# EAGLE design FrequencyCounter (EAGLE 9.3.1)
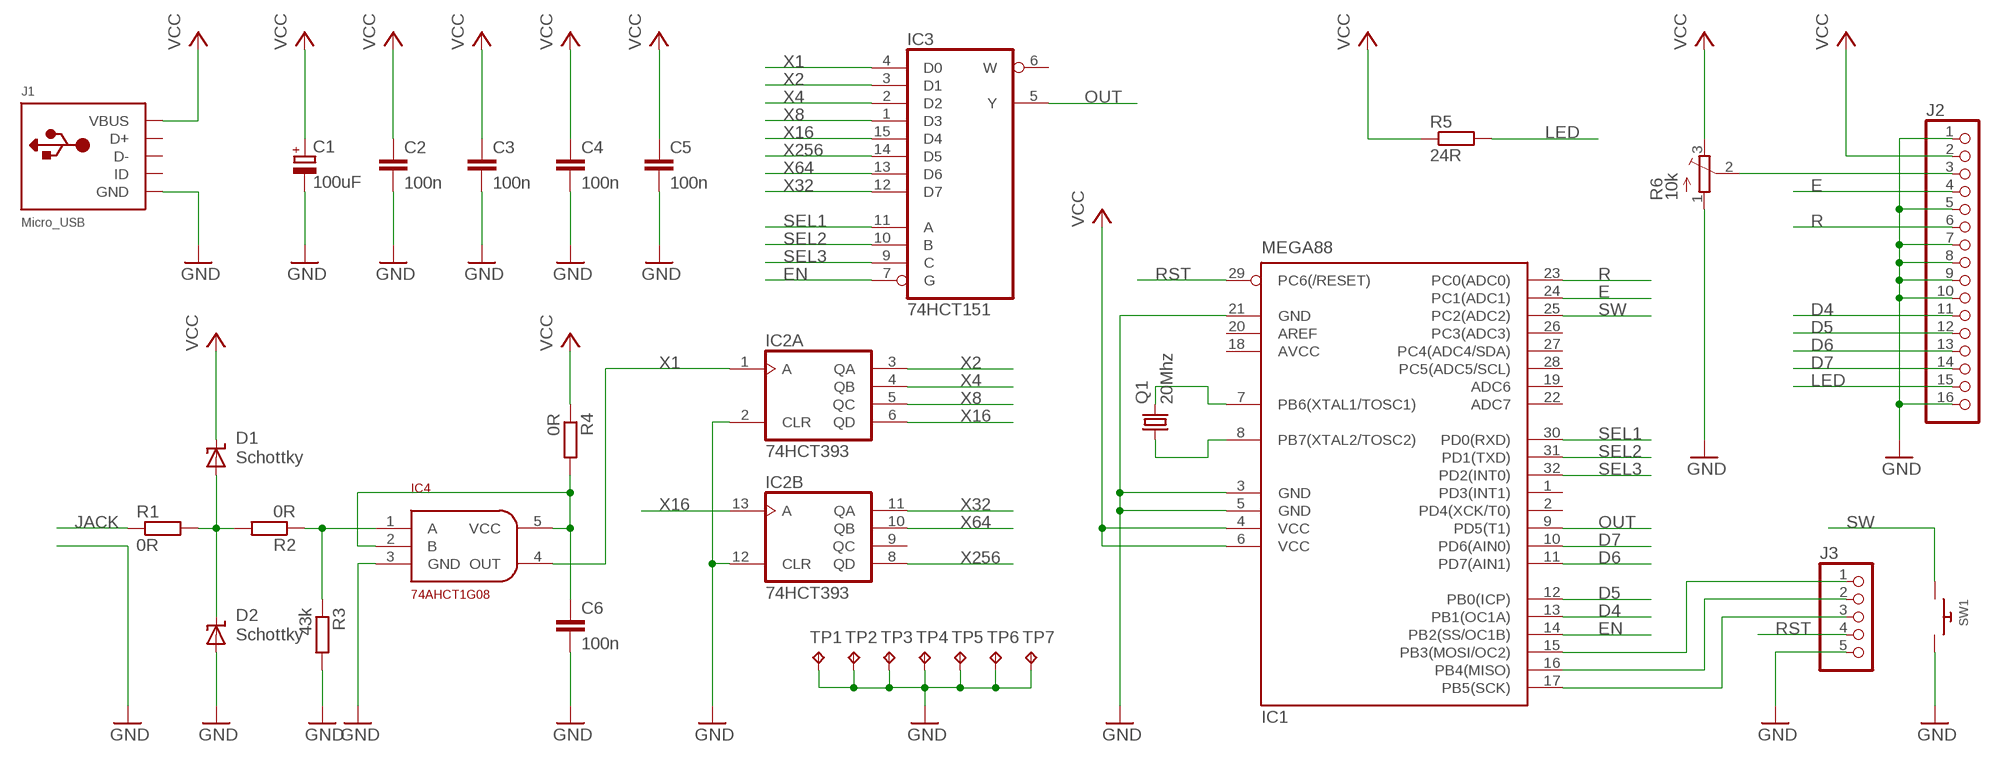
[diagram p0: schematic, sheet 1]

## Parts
C1  100uF  CPOL-EU153CLV-0605  [153CLV-0605]
C2  100n  C-EUC1206  [C1206]
C3  100n  C-EUC1206  [C1206]
C4  100n  C-EUC1206  [C1206]
C5  100n  C-EUC1206  [C1206]
C6  100n  C-EUC1206  [C1206]
D1  Schottky  SUPPRESSOR-SMBJ  [SMBJ]
D2  Schottky  SUPPRESSOR-SMBJ  [SMBJ]
IC1  MEGA88  MEGA8-AI  [TQFP32-08]
IC2  74HCT393  74AC393D  [SO14]
IC3  74HCT151  74AC151D  [SO16]
IC4  74AHCT1G08  [SOT-23-5]
J1  Micro_USB  USBMINIB  [USB-MINIB]
J2  PINHD-1X16  [1X16]
J3  PINHD-1X5  [1X05]
Q1  20Mhz  CSM-7X-DU  [CSM-7X-DU]
R1  0R  R-EU_M1206  [M1206]
R2  0R  R-EU_M1206  [M1206]
R3  43k  R-EU_M1206  [M1206]
R4  0R  R-EU_M1206  [M1206]
R5  24R  R-EU_M1206  [M1206]
R6  10k  TRIM_EU-3223G  [3223G]
SW1  SWITCH_PUSHBUTTONC&K_KSS  [BTN_CK_KSS]
TP1  TPPAD1-13  [P1-13]
TP2  TPPAD1-13  [P1-13]
TP3  TPPAD1-13  [P1-13]
TP4  TPPAD1-13  [P1-13]
TP5  TPPAD1-13  [P1-13]
TP6  TPPAD1-13  [P1-13]
TP7  TPPAD1-13  [P1-13]

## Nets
D4: IC1.13(PB1(OC1A)) J2.11
D5: IC1.12(PB0(ICP)) J2.12
D6: IC1.11(PD7(AIN1)) J2.13
D7: IC1.10(PD6(AIN0)) J2.14
E: IC1.24(PC1(ADC1)) J2.4
EN: IC1.14(PB2(SS/OC1B)) IC3.7(G)
GND: C1.- C2.2 C3.2 C4.2 C5.2 C6.2 D2.A IC1.3(GND) IC1.5(GND) IC1.21(GND) IC2.2(A:CLR) IC2.12(B:CLR) IC4.3(GND) J1.GND J2.1 J2.5 J2.7 J2.8 J2.9 J2.10 J2.16 J3.5 R3.2 R6.1(A) SW1.P$2 TP1.TP TP2.TP TP3.TP TP4.TP TP5.TP TP6.TP TP7.TP
JACK: R1.1
LED: J2.15 R5.2
N$1: IC1.17(PB5(SCK)) J3.3
N$2: D1.A D2.C R1.2 R2.2
N$3: IC4.1(A) R2.1 R3.1
N$4: IC1.16(PB4(MISO)) J3.2
N$5: IC1.15(PB3(MOSI/OC2)) J3.1
N$6: IC1.8(PB7(XTAL2/TOSC2)) Q1.1
N$7: IC1.7(PB6(XTAL1/TOSC1)) Q1.2
N$8: J2.3 R6.2(S)
N$10: C6.1 IC4.2(B) IC4.5(VCC) R4.2
OUT: IC1.9(PD5(T1)) IC3.5(Y)
R: IC1.23(PC0(ADC0)) J2.6
RST: IC1.29(PC6(/RESET)) J3.4
SEL1: IC1.30(PD0(RXD)) IC3.11(A)
SEL2: IC1.31(PD1(TXD)) IC3.10(B)
SEL3: IC1.32(PD2(INT0)) IC3.9(C)
SW: IC1.25(PC2(ADC2)) SW1.P$1
VCC: C1.+ C2.1 C3.1 C4.1 C5.1 D1.C IC1.4(VCC) IC1.6(VCC) J1.VBUS J2.2 R4.1 R5.1 R6.3(E)
X1: IC2.1(A:A) IC3.4(D0) IC4.4(OUT)
X2: IC2.3(A:QA) IC3.3(D1)
X4: IC2.4(A:QB) IC3.2(D2)
X8: IC2.5(A:QC) IC3.1(D3)
X16: IC2.6(A:QD) IC2.13(B:A) IC3.15(D4)
X32: IC2.11(B:QA) IC3.12(D7)
X64: IC2.10(B:QB) IC3.13(D6)
X256: IC2.8(B:QD) IC3.14(D5)
Unconnected: IC1.1(PD3(INT1)) IC1.2(PD4(XCK/T0)) IC1.19(ADC6) IC1.20(AREF) IC1.22(ADC7) IC1.26(PC3(ADC3)) IC1.27(PC4(ADC4/SDA)) IC1.28(PC5(ADC5/SCL)) IC2.9(B:QC) IC3.6(W) J1.D+ J1.D- J1.ID

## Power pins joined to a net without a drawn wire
AVCC: IC1.18(AVCC)
GND: IC2.7(P:GND) IC3.8(GND)
VCC: IC2.14(P:VCC) IC3.16(VCC)

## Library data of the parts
C1 = rcl:CPOL-EU: POLARIZED CAPACITOR, European symbol
C2-C6 = rcl:C-EU: CAPACITOR, European symbol
D1 D2 = diode:SUPPRESSOR-: Suppressor diode
IC1 = atmel:MEGA8: MICROCONTROLLER 8 Kbytes FLASH, 1 kbytes SRAM, 512 bytes EEPROM, USART, 6-channel 10 bit ADC, 2-channel 8 bit ADC Pin compatible with Atmega48, ATMega88, ATMega168 Source: avr.lbr; MPN: ATMEGA8-16AU; OC_FARNELL: 9171371; OC_NEWARK: 73M8863
IC2 = 74xx-eu:74*393: Dual 4-bit decade and binary COUNTER
IC3 = 74xx-eu:74*151: Data SELECTOR/MULTIPLEXER
IC4 = 0stepanovsky:74AHCT1G08
J1 = adafruit:USB: USB Connectors USBMINIB - Surface Mount Female Mini-B USB Connector 4UConnector: 06564 By microbuilder.eu Thru-hole RA Female Mini-B USB Connector 4UConnector: 18732 By ladyada.net
J2 = pinhead:PINHD-1X16: PIN HEADER
J3 = pinhead:PINHD-1X5: PIN HEADER
Q1 = crystal:CSM-7X-DU: SMD CRYSTAL; OC_FARNELL: unknown; OC_NEWARK: unknown
R1-R5 = resistor:R-EU_: RESISTOR, European symbol
R6 = pot:TRIM_EU-: POTENTIOMETER
SW1 = adafruit:SWITCH_PUSHBUTTON: Buttons
TP1-TP7 = testpad:TP: Test pad

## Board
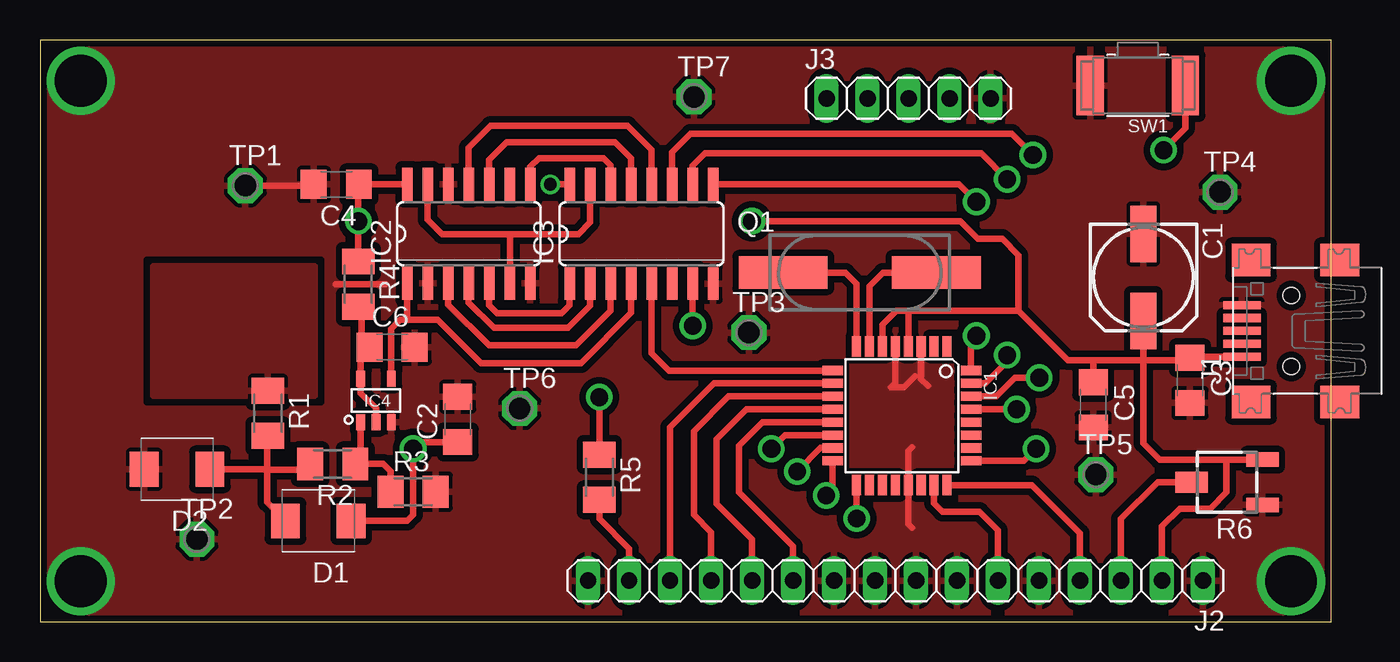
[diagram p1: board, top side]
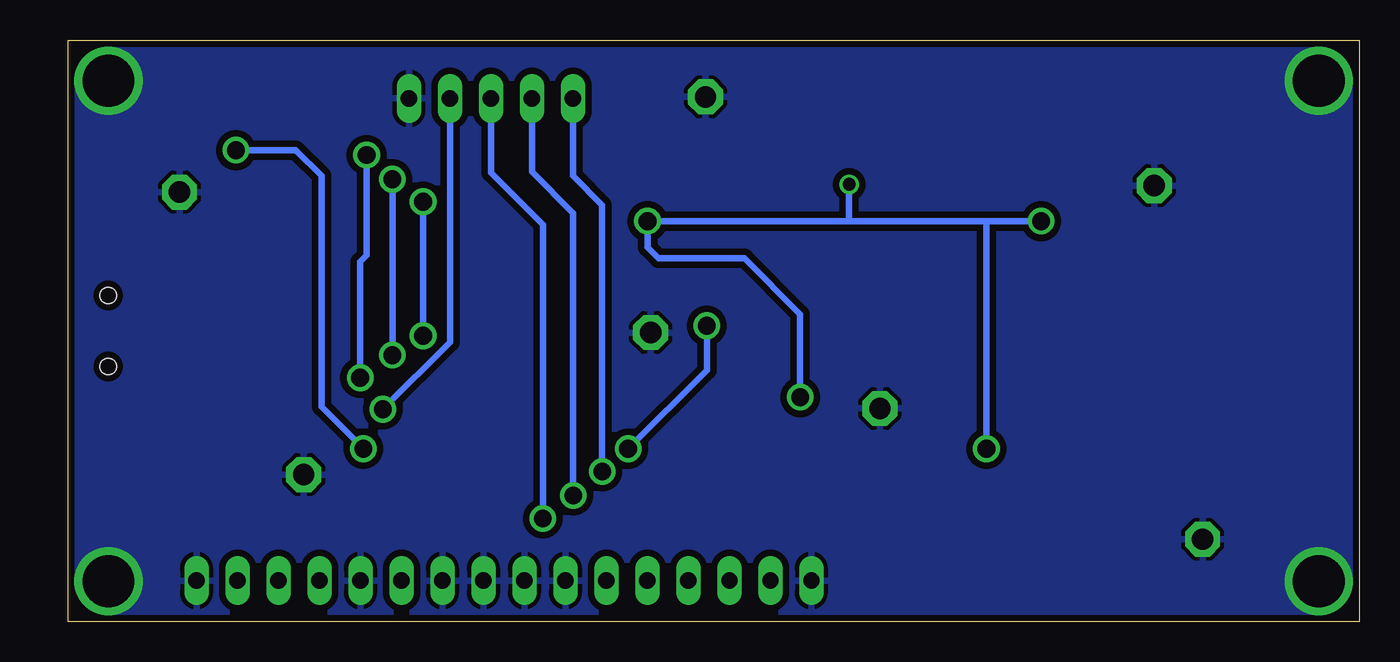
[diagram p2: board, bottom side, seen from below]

Size 80 x 36 mm. Coordinates in mm from the lower left corner, seen from the top.
Outline: 0,0 80,0 80,36 0,36 0,0
Copper layers (1*16): Top 0.035mm / dielectric 1.5mm / Bottom 0.035mm
Design rules "default *": minimum track width 10mil, minimum drill 24mil, track to track 8mil, track to pad 8mil, pad to pad 8mil, via to via 8mil, smd to smd 8mil, copper to edge 10mil, drill to drill 8mil, minimum pad ring 10mil, minimum via ring 8mil, stop-mask expansion 4mil, vias tented up to drill 0mil, thermal gap 10mil

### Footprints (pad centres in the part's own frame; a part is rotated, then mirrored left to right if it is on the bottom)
153CLV-0605 = smd 3.5 x 1.6: + 2.7,0; - -2.7,0
C1206 = smd 1.6 x 1.8: 1 -1.4,0; 2 1.4,0
SMBJ = smd 1.78 x 2.16: A 2.04,0; C -2.03,0
TQFP32-08 = smd 1.27 x 0.559: 1 -4.293,2.8; 2 -4.293,2; 3 -4.293,1.2; 4 -4.293,0.4; 5 -4.293,-0.4; 6 -4.293,-1.2; 7 -4.293,-2; 8 -4.293,-2.8; 17 4.293,-2.8; 18 4.293,-2; 19 4.293,-1.2; 20 4.293,-0.4; 21 4.293,0.4; 22 4.293,1.2; 23 4.293,2; 24 4.293,2.8 | smd 0.559 x 1.27: 9 -2.8,-4.293; 10 -2,-4.293; 11 -1.2,-4.293; 12 -0.4,-4.293; 13 0.4,-4.293; 14 1.2,-4.293; 15 2,-4.293; 16 2.8,-4.293; 25 2.8,4.293; 26 2,4.293; 27 1.2,4.293; 28 0.4,4.293; 29 -0.4,4.293; 30 -1.2,4.293; 31 -2,4.293; 32 -2.8,4.293
SO14 = smd 0.66 x 2.032: 1 -3.81,-3.073; 2 -2.54,-3.073; 3 -1.27,-3.073; 4 0,-3.073; 5 1.27,-3.073; 6 2.54,-3.073; 7 3.81,-3.073; 8 3.81,3.073; 9 2.54,3.073; 10 1.27,3.073; 11 0,3.073; 12 -1.27,3.073; 13 -2.54,3.073; 14 -3.81,3.073
SO16 = smd 0.66 x 2.032: 1 -4.445,-3.073; 2 -3.175,-3.073; 3 -1.905,-3.073; 4 -0.635,-3.073; 5 0.635,-3.073; 6 1.905,-3.073; 7 3.175,-3.073; 8 4.445,-3.073; 9 4.445,3.073; 10 3.175,3.073; 11 1.905,3.073; 12 0.635,3.073; 13 -0.635,3.073; 14 -1.905,3.073; 15 -3.175,3.073; 16 -4.445,3.073
SOT-23-5 = smd 1 x 0.55: 1 -1.35,0.95; 2 -1.35,0; 3 -1.35,-0.95; 4 1.35,-0.95; 5 1.35,0.95
USB-MINIB = smd 0.5 x 2.308: D+ 0,4.064; D- -0.8,4.064; GND 1.6,4.064; ID 0.8,4.064; VBUS -1.6,4.064 | smd 2 x 2.4: GND1 -4.4,-2; GND2 -4.4,3.5; GND3 4.4,3.5; GND4 4.4,-2 | hole 1: -2.2,1; 2.2,1
1X16 = drill 1.016 long: 1 -19.05,0; 2 -16.51,0; 3 -13.97,0; 4 -11.43,0; 5 -8.89,0; 6 -6.35,0; 7 -3.81,0; 8 -1.27,0; 9 1.27,0; 10 3.81,0; 11 6.35,0; 12 8.89,0; 13 11.43,0; 14 13.97,0; 15 16.51,0; 16 19.05,0
1X05 = drill 1.016 long: 1 -5.08,0; 2 -2.54,0; 3 0,0; 4 2.54,0; 5 5.08,0
CSM-7X-DU = smd 5.5 x 2: 1 -4.75,0; 2 4.75,0
M1206 = smd 1.6 x 2: 1 -1.4,0; 2 1.4,0
3223G = smd 2 x 0.9: 1 -2.2,1.4; 3 -2.2,-1.4 | smd 2 x 1.3: 2 2.2,0
BTN_CK_KSS = smd 1.7 x 3.7: P$1 -2.95,0; P$2 2.95,0
P1-13 = drill 1.321 pad 2.159 octagon: TP 0,0

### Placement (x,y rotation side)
C1  68.35,21.32 270 top
C2  25.86,12.52 90 top
C3  71.24,14.94 270 top
C4  18.34,27.08 180 top
C5  65.24,13.42 270 top
C6  21.8,17 0 top
D1  17.23,6.23 180 top
D2  8.48,9.43 180 top
IC1  53.38,12.75 270 top
IC2  26.55,24.02 0 top
IC3  37.25,24.01 0 top
IC4  20.8,13.7 90 top
J1  78.52,18 90 top
J2  52.99,2.54 180 top
J3  53.8,32.4 0 top
Q1  50.78,21.62 0 top
R1  14.1,12.9 270 top
R2  18.12,9.76 180 top
R3  23.1,8.04 0 top
R4  19.7,20.9 270 top
R5  34.64,8.94 270 top
R6  73.53,8.63 180 top
SW1  68,33.2 180 top
TP1  12.7,27 0 top
TP2  9.7,5.1 0 top
TP3  43.9,17.9 0 top
TP4  73.1,26.6 0 top
TP5  65.4,9.1 0 top
TP6  29.7,13.2 0 top
TP7  40.5,32.5 0 top

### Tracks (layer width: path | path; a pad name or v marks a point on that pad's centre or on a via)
D4
  Top 0.406: J2.11 46.64,4.66 43.3,8 43.3,10.9 44.75,12.35 IC1.13
D5
  Top 0.406: J2.12 44.1,5.1 41.9,7.3 41.9,11.3 43.75,13.15 IC1.12
D6
  Top 0.406: J2.13 41.56,5.54 40.5,6.6 40.5,11.8 42.65,13.95 IC1.11
D7
  Top 0.406: J2.14 39.02,12.02 41.75,14.75 IC1.10
E
  Top 0.406: J2.4 64.42,5.48 61.44,8.46 IC1.24
EN  (via drill 1.1)
  Top 0.406: IC1.14 46.15,11.55 v45.3,10.7 | v40.42,18.32 IC3.7
  Bottom 0.406: v45.3,10.7 40.42,15.57 v40.42,18.32
GND  (via drill 3.2)
  Top 0.406: 18.3,20.9 21.4,20.9 | 54,5.8 53.78,6.02 IC1.21 53.78,10.58 54,10.8 | IC1.5 52.98,14.78 52.7,14.5 53.5,14.5 54.2,15.2 | IC1.3 54.58,15.02 55,14.6 | TP1.TP 16.86,27 C4.2
  other vias: 2.5,33.5 77.5,33.5 77.5,2.5 2.5,2.5
  pour Top (isolate 0.406, rank 2): 3,35.5 77,35.5 79.5,33 79.5,3 77,0.5 3,0.5 0.5,3 0.5,33
  pour Bottom (isolate 0.406): 0.5,33 3,35.5 77,35.5 79.5,33 79.5,3 77,0.5 3,0.5 0.5,3
JACK
  pour Top: 7,22 17,22 17,14 7,14
LED
  Top 0.406: J2.15 36.48,4.52 34.64,6.36 R5.2
N$1  (via drill 1.1)
  Top 0.406: IC1.17 v50.58,6.38
  Bottom 0.406: J3.3 53.8,27.8 50.58,24.58 v50.58,6.38
N$2
  Top 0.406: D1.A 14.04,7.38 14.04,9.4 | D2.C 14.01,9.43 14.04,9.4 | 14.04,9.4 14.04,11.44 R1.2 | 14.04,9.4 16.36,9.4 R2.2
N$3
  Top 0.406: IC4.1 19.85,10.09 R2.1 21.24,9.76 21.7,9.3 R3.1
N$4  (via drill 1.1)
  Top 0.406: IC1.16 49.09,8.19 v48.7,7.8
  Bottom 0.406: J3.2 51.26,27.86 48.7,25.3 v48.7,7.8
N$5  (via drill 1.1)
  Top 0.406: IC1.15 48.35,10.75 v46.9,9.3
  Bottom 0.406: J3.1 48.72,27.62 46.9,25.8 v46.9,9.3
N$6
  Top 0.406: IC1.8 50.58,20.92 49.88,21.62 Q1.1
N$7
  Top 0.406: IC1.7 51.38,20.78 52.22,21.62 Q1.2
N$8
  Top 0.406: 66.93,2.57 J2.3 66.96,6.36 69.23,8.63 R6.2
N$10
  Top 0.406: IC4.2 20.8,13.2 19.85,14.15 IC4.5 19.85,16.45 C6.1 19.9,17.5 19.9,19.3 R4.2
OUT
  Top 0.406: IC1.9 38.95,15.55 37.88,16.61 IC3.5
R
  Top 0.406: IC1.23 55.38,7.32 55.9,6.8 58.2,6.8 59.34,5.66 J2.6
RST  (via drill 1.1)
  Top 0.406: IC1.29 v60.5,13.15
  Bottom 0.406: v60.5,13.15 56.34,17.31 J3.4
SEL1  (via drill 1.1)
  Top 0.406: IC3.11 39.16,29.05 40.3,30.2 60.2,30.2 v61.5,28.9 | IC1.30 59.25,13.95 60.4,15.1 v61.9,15.1
  Bottom 0.406: v61.9,15.1 61.9,22.3 61.5,22.7 v61.5,28.9
SEL2  (via drill 1.1)
  Top 0.406: IC3.10 40.42,28.23 41.2,29 58.3,29 v59.9,27.4 | IC1.31 58.55,14.75 59.9,16.1 v59.9,16.5
  Bottom 0.406: v59.9,27.4 v59.9,16.5
SEL3  (via drill 1.1)
  Top 0.406: IC3.9 56.92,27.08 v58,26 | IC1.32 57.67,17.37 v58,17.7
  Bottom 0.406: v58,26 v58,17.7
SW  (via drill 1.1)
  Top 0.406: SW1.P$1 70.95,30.55 v69.6,29.2 | v61.7,10.7 60.95,9.95 IC1.25
  Bottom 0.406: v69.6,29.2 65.9,29.2 64.3,27.6 64.3,13.3 v61.7,10.7
VCC  (via drill 0.8, 1.1)
  Top 0.406: IC1.6 52.18,18.38 53.06,19.26 53.8,19.26 | 53.8,19.26 60.6,19.26 | IC1.4 53.78,19.24 53.8,19.26 | IC2.14 19.75,27.09 C4.1 19.7,27.04 v19.7,24.8 R4.1 | J2.2 69.5,5.9 70.6,7 72.5,7 73.5,8 73.5,10.03 | R6.3 73.5,10.03 | 73.5,10.03 69.37,10.03 68.35,11.05 68.35,16.2 | v44.1,24.8 57,24.8 58.1,23.7 59.6,23.7 60.6,22.7 60.6,19.26 | R5.1 v34.64,13.9 | D1.C 22.73,6.23 23.1,6.6 v23.1,10.7 23.52,11.12 C2.1 | IC3.16 v31.6,27.08 | J1.VBUS 71.24,16.4 | 71.24,16.4 C3.1 | 68.35,16.2 C1.+ | 71.24,16.4 71.04,16.2 68.35,16.2 | 68.35,16.2 65.3,16.2 | 65.3,16.2 63.66,16.2 60.6,19.26 | C5.1 65.24,16.14 65.3,16.2
  Bottom 0.406: 31.6,24.8 v44.1,24.8 44.1,23.2 43.4,22.5 38.1,22.5 34.64,19.04 v34.64,13.9 | 31.6,24.8 23.1,24.8 | 23.1,24.8 v19.7,24.8 | 23.1,24.8 v23.1,10.7 | v31.6,27.08 31.6,24.8
X1
  Top 0.406: IC3.4 36.62,19.11 33.5,16 27.3,16 24.6,18.7 22.74,18.7 | IC2.1 22.74,18.7 | 22.74,18.7 22.3,18.7 21.75,18.15 IC4.4
X2
  Top 0.406: IC2.3 25.28,19.62 27.8,17.1 33.2,17.1 35.34,19.25 IC3.3
X4
  Top 0.406: IC2.4 26.55,19.75 28.1,18.2 32.7,18.2 34.08,19.57 IC3.2
X8
  Top 0.406: IC2.5 27.82,19.58 28.3,19.1 32.3,19.1 32.8,19.61 IC3.1
X16
  Top 0.406: IC3.15 34.08,24.73 33.35,24 29.1,24 | IC2.6 29.1,24 | 29.1,24 24.9,24 24.01,24.89 IC2.13
X32
  Top 0.406: IC3.12 37.88,29.21 36.4,30.7 27.9,30.7 26.55,29.35 IC2.11
X64
  Top 0.406: IC3.13 36.62,28.68 35.6,29.7 28.9,29.7 27.82,28.62 IC2.10
X256
  Top 0.406: IC3.14 35.34,28.25 34.9,28.7 30.9,28.7 30.36,28.16 IC2.8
